(* Logix 5000 DataType export SD_Control; software revision 20.01 *)

TYPE SD_Control :   // Smart drive 控制数据
STRUCT
   MotorFW : BOOL;   // 电机正传
   MotorRVS : BOOL;   // 电机反转
   Reset : BOOL;   // 系统复位
   Output1 : BOOL;   // 输出1
   Output2 : BOOL;   // 输出2
   Output3 : BOOL;   // 输出3
   Output4 : BOOL;   // 输出4
   LocalEnable : BOOL;   // 转速,停止由smart drive内部控制
   Speed : INT;   // 运行速度 10000对应50HZ
   AccelerTime : INT;   // 加速时间
   DecelerTime : INT;   // 减速时间
END_STRUCT
END_TYPE
